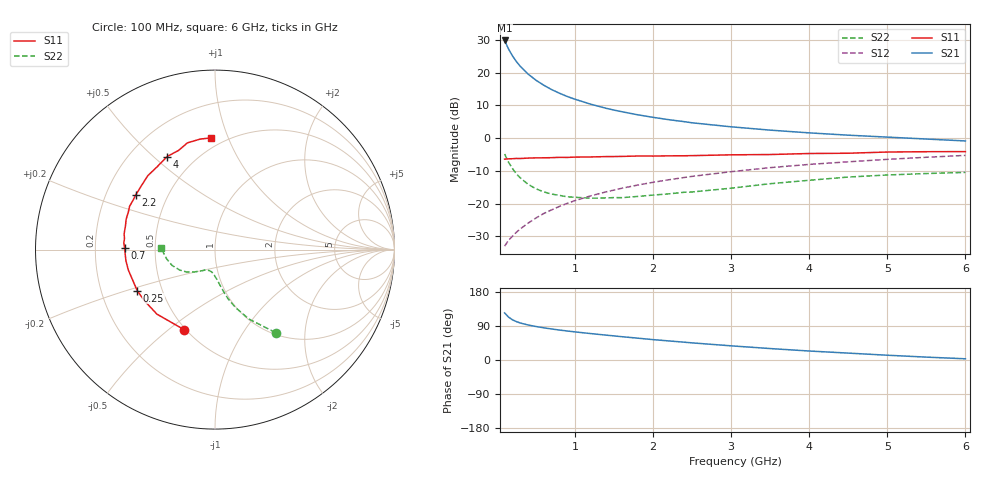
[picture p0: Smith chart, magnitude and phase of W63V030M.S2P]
! SIEMENS Small Signal Semiconductors
! BFR193W
! Si NPN RF Bipolar Junction Transistor in SOT323
! VCE = 3 V  IC = 30 mA
! Common Emitter S-Parameters:  September  1992
# GHz  S  MA  R  50
!  f  S11  S21  S12  S22
! GHz  MAG  ANG  MAG  ANG  MAG  ANG  MAG  ANG
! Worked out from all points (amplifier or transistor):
!   28 points, 100 MHz to 6 GHz, reference 50 ohm
!   highest |S21| = 29.9 dB at 100 MHz (marker M1)
!   |S21| within 3 dB of that: start of sweep to 159.8 MHz
!   unconditionally stable (mu >= 1): 626.1 MHz to 2.488 GHz
!   at 300 MHz: K = 0.85, MSG = 24.8 dB, |S12| = -27.7 dB
!   at 1.5 GHz: K = 1.03, MAG = 11.1 dB, |S12| = -15.9 dB
!   at 6 GHz: K = 0.92, MSG = 2.2 dB, |S12| = -5.3 dB
!   lowest NFmin = 1.90 dB at 450 MHz
!   S11 on the Smith chart (normalised r, x): 100 MHz: 0.49, -0.57; 250 MHz: 0.36, -0.22; 700 MHz: 0.33, +0.01; 2.2 GHz: 0.33, +0.28; 4 GHz: 0.35, +0.55; 6 GHz: 0.43, +0.87
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0.1  0.4783 -111.0  31.09 124.3  0.0224 58.8  0.5723 -53.9
0.15  0.4837 -132.0  23.07 113.2  0.0275 57.7  0.43 -64.0
0.2  0.4855 -144.0  18.13 106.1  0.0318 59.0  0.3446 -70.3
0.25  0.49 -152.2  14.84 101.4  0.0365 61.0  0.2855 -75.0
0.3  0.4887 -158.3  12.55 97.7  0.0411 62.8  0.2483 -77.7
0.4  0.4963 -166.9  9.54 92.4  0.0503 65.9  0.1976 -82.3
0.5  0.5 -172.7  7.7 88.4  0.0602 67.7  0.1688 -85.8
0.6  0.5011 -177.1  6.453 85.0  0.0705 68.8  0.1514 -89.6
0.7  0.5035 179.2  5.535 81.9  0.0802 69.6  0.1402 -92.1
0.8  0.5094 175.7  4.873 79.1  0.0905 70.0  0.1337 -95.1
0.9  0.5081 173.0  4.341 76.6  0.1008 70.0  0.1273 -97.2
1  0.5139 170.2  3.939 74.2  0.1111 70.1  0.1251 -99.4
1.2  0.5163 165.0  3.309 69.8  0.1312 69.5  0.1211 -105.0
1.4  0.5231 161.1  2.861 65.6  0.1513 68.7  0.1221 -109.2
1.6  0.5263 156.5  2.537 61.5  0.1716 67.7  0.1233 -113.3
2.2  0.537 145.2  1.918 50.4  0.2312 63.7  0.1409 -122.6
3  0.5565 132.3  1.491 37.4  0.3077 57.4  0.1722 -133.6
3.5  0.5626 125.1  1.327 30.2  0.3547 53.1  0.2016 -141.8
4  0.583 117.2  1.205 23.7  0.3973 48.7  0.2274 -150.0
4.5  0.5888 110.1  1.111 18.2  0.4355 44.4  0.2548 -159.7
5.5  0.6212 97.7  0.97 7.6  0.5108 35.9  0.2882 -176.7
6  0.6232 91.9  0.907 3.2  0.5457 31.5  0.3001 178.5
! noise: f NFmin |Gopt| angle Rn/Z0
0.45  1.9  0.4  180  0.09
0.9  1.95  0.43  -173  0.11
1.8  2.4  0.58  -144  0.24
